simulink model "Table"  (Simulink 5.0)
settings: Solver=FixedStepDiscrete  SolverMode=SingleTasking  StartTime=0.0  StopTime=inf  FixedStep=samplePeriod  RelTol=1e-3  AbsTol=1e-6
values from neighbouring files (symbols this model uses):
  accelCalib = ones(1, size(ra_t, 2)) * 7848.0    [TableInit.m]
  actParamsX = [bulkModulus    * pressCanon,    [TableInit.m]
  actParamsY = [bulkModulus    * pressCanon,    [TableInit.m]
  actParamsZ = [bulkModulus    * pressCanon,    [TableInit.m]
  aHome = zeros(1, nAct)    [TableInit.m]    (also in displA2T.m = positT2A([0, 0, 0, 0, 0, 0], h); displT2A.m = positT2A([0, 0, 0, 0, 0, 0], h))
  bal = [[ 1 -1 -1  1  0  0  0  0]    [TableInit.m]
  displCalib = [300.0 300.0 300.0 300.0 250.0 250.0 250.0 250.0]    [TableInit.m]
  ea_t = zeros(3, nAcc)    [TableInit.m]
  flowCanon = 63090.2    [TableInit.m]    (also in initialize.m)
  forceCalib = [366.5 366.5 366.5 366.5 366.5 366.5 366.5 366.5]    [TableInit.m]
  gasConstant = 1.8    [TableInit.m]    (also in initialize.m)
  gee = 0    [TableInit.m]    (also in initialize.m = geeCanon / linAccelCanon * ~isempty(find(dof==3)))
  inertia = [Ixx 0 0; 0 Iyy 0; 0 0 Izz]    [TableInit.m]    (also in initialize.m = inertia + inertiaP2Q([0 0 0], massA(i), cgA(:,i)-cg,  						)
  inertiaCanon = 0.1130    (= 0.113)    [TableInit.m]    (also in initialize.m = 0.00029264264)
  linAccelCanon = 9.8    [TableInit.m]    (also in accelA2T.m = h(11); accelT2A.m = h(11); Test.m = 9800; initialize.m = 9810)
  linVelocCanon = 10.0    (= 10)    [TableInit.m]    (also in Test.m; initialize.m = 1000)
  mass = 17300    [TableInit.m]    (also in initialize.m = ones(3, 1) * (sum(massA) + massT + massS))
  massCanon = 0.4535924e-06    (= 4.535924e-07)    [TableInit.m]    (also in initialize.m)
  maxDispl = zeros(1, nAct)    [TableInit.m]    (also in initialize.m = max(abs(maxDispl), abs(minDispl)))
  maxOilVolume = volume * (1 - (precharge/supplyPress)^(1/gasConstant))    (= 316.850998915)    [TableInit.m]
  precharge = 1916    [TableInit.m]    (also in initialize.m = 2000)
  pumpFlow = 1.0e10    (= 10000000000)    [TableInit.m]    (also in initialize.m)
  ra_t = [-1600.00   233.10  -233.10  1600.00 -1000.00  1000.00 -1000.00  1000.00        0    [TableInit.m]    (also in accelA2T.m = [  0   0   0 -h7  h7   0 -h7 -h7  h7  h7   0;          -h7  ; accelT2A.m = [  0   0   0 -h7  h7   0 -h7 -h7  h7  h7   0;          -h7  )
  rb_w = [-1525.00  3683.70 -3683.70  1525.00 -1000.00  1000.00 -1000.00  1000.00    [TableInit.m]    (also in positT2A.m = [-h1 -h5  h5  h1 -h1 -h1  h1  h1;           h5 -h1  h1 -h5  ; animation.m = self.R * rb_w)
  returnPress = 50    [TableInit.m]    (also in initialize.m)
  rgt = -rtg    [TableInit.m]
  rotAccelCanon = 1    [TableInit.m]    (also in accelA2T.m = h(14); accelT2A.m = h(14); Test.m; initialize.m = 0.0174532925199)
  rotForceCanon = 1000    [TableInit.m]    (also in forceA2T.m = h(15); Test.m; initialize.m)
  rotVelocCanon = 1    [TableInit.m]    (also in accelA2T.m = h(13); accelT2A.m = h(13); Test.m; initialize.m = 0.0174532925199)
  rt_t = [-1525.00  1214.70 -1214.70  1525.00 -1000.00  1000.00 -1000.00  1000.00    [TableInit.m]    (also in positT2A.m = [-h1    -h4-sh  h4+sh  h1    -h1    -h1     h1     h1;      )
  rtg = [0 0 cg]    [TableInit.m]    (also in initialize.m = cg)
  rtx_t = [rt_t topPlane.topLeft(:)  topPlane.topRight(:)                        topPlane.botRight(:) topPlane.botLeft(:)                         midPlane.topLeft(:)  midPlane.topRight(:)                        midPlane.botRight(:) midPlane.botLeft(:)                         botPlane.topLeft(:)  botPlane.topRight(:)                        botPlane.botRight(:) botPlane.botLeft(:)]    [TableInit.m]
  samplePeriod = 1/1024    (= 0.0009765625)    [TableInit.m]    (also in viewer.m = eval(getHeaderValue(header, 'DELTA_T')); initialize.m = 0.00048828125)
  volume = 1437    [TableInit.m]    (also in quake.m = volume / 231.0; initialize.m = 160)
  volumeCanon = 3785412.0    (= 3785412)    [TableInit.m]    (also in initialize.m)
undefined symbols (not defined in the file or in its folder): magnitude
libraries: aerospace x41, simulink x19, simulink_extras x1

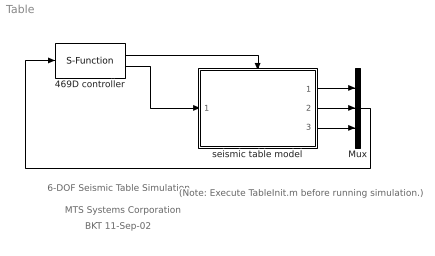
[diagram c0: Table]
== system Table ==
  note: BKT 11-Sep-02
  note: MTS Systems Corporation
  note: 6-DOF Seismic Table Simulation
  note: (Note: Execute TableInit.m before running simulation.)
  469D controller : S-Function  FunctionName=mtsConnect  Parameters='127.0.0.1',5002,nAct+nAct+nAcc,nAct
  Mux : Mux  Inputs=3
  seismic table model : Subsystem  TreatAsAtomicUnit=on
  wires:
  seismic table model/1(displ) -> Mux/1
  seismic table model/2(force) -> Mux/2
  seismic table model/3(accel) -> Mux/3
  Mux/1 -> 469D controller/1
  469D controller/2 -> seismic table model/1(valve cmd)
  469D controller/1 -> seismic table model/Trigger

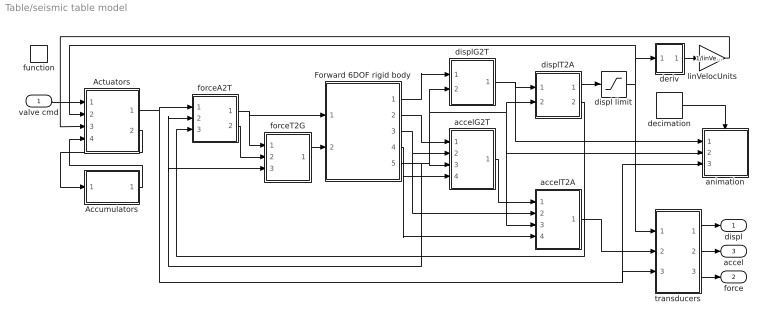
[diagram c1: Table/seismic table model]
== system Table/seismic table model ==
  valve cmd : Inport
  function : TriggerPort  TriggerType=function-call
  Accumulators : Subsystem
  Actuators : Subsystem
  Forward 6DOF rigid body : Subsystem
  accelG2T : Subsystem
  accelT2A : Subsystem
  animation : Subsystem  TreatAsAtomicUnit=on  mask{type=2, azim=-37.5, elev=15}
      mask prompts: type "Drawing type (0: none, 1: wire frame, 2: solid)"; azim "View azimuth (degrees)"; elev "View elevation (degrees)"
  decimation : DiscretePulseGenerator  Period=64  SampleTime=-1
  deriv : Subsystem  mask{T=samplePeriod}
      mask prompts: T "Sample period (sec)"
  displ limit : Saturate  UpperLimit=maxDispl(:)  LowerLimit=-maxDispl(:)
  displG2T : Subsystem
  displT2A : Subsystem
  forceA2T : Subsystem
  forceT2G : Subsystem
  linVelocUnits : Gain  Gain=1/linVelocCanon
  transducers : Subsystem
  displ : Outport
  force : Outport  Port=2
  accel : Outport  Port=3
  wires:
  valve cmd/1 -> Actuators/1(cmds)
  displT2A/1(out) -> displ limit/1
  deriv/1(out) -> linVelocUnits/1
  displT2A/2(dir) -> forceA2T/3(dir)
  Actuators/1(force) -> forceA2T/1(inp), transducers/3(force), animation/3(Fact)
  forceA2T/1(xyz) -> forceT2G/1(xyz), Forward 6DOF rigid body/1(Fxyz)
  displG2T/1(out) -> displT2A/1(xyz), animation/1(xyz)
  Forward 6DOF rigid body/5(DCM) -> displT2A/2(DCM), accelT2A/3(DCM), animation/2(DCM), displG2T/2(DCM), accelG2T/3(DCM), forceA2T/2(DCM), forceT2G/3(DCM)
  accelG2T/1(out) -> accelT2A/1(xyz)
  forceA2T/2(rpw) -> forceT2G/2(rpw)
  forceT2G/1(out) -> Forward 6DOF rigid body/2(Mxyz)
  displ limit/1 -> Actuators/2(displ), deriv/1(inp), transducers/1(displ)
  Forward 6DOF rigid body/1(xyz) -> displG2T/1(xyz)
  Forward 6DOF rigid body/4(rot veloc) -> accelT2A/4(rot veloc), accelG2T/4(rot veloc)
  Forward 6DOF rigid body/3(rot accel) -> accelT2A/2(rpw), accelG2T/2(rpw)
  Forward 6DOF rigid body/2(lin accel) -> accelG2T/1(xyz)
  linVelocUnits/1 -> Actuators/3(veloc)
  Actuators/2(flow) -> Accumulators/1(flow)
  Accumulators/1(press) -> Actuators/4(press)
  accelT2A/1(out) -> transducers/2(accel)
  transducers/1(out1) -> displ/1
  transducers/2(out2) -> accel/1
  transducers/3(out3) -> force/1
  decimation/1 -> animation/Trigger

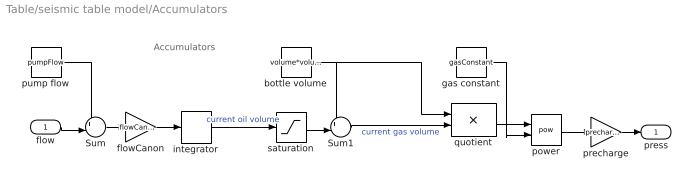
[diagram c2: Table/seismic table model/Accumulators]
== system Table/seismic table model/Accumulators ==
  note: Accumulators
  flow : Inport
  Sum : Sum  Inputs=+-|
  Sum1 : Sum  Inputs=+-|
  bottle volume : Constant  Value=volume*volumeCanon
  flowCanon : Gain  Gain=flowCanon
  gas constant : Constant  Value=gasConstant
  integrator : DiscreteIntegrator  InitialCondition=volume * (1 - (precharge/3000)^(1/gasConstant)) * 231  SampleTime=-1
  power : Math  Operator=pow
  precharge : Gain  Gain=precharge
  pump flow : Constant  Value=pumpFlow
  quotient : Product  Inputs=*/
  saturation : Saturate  UpperLimit=maxOilVolume*volumeCanon  LowerLimit=0
  press : Outport
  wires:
  pump flow/1 -> Sum/1
  Sum/1 -> flowCanon/1
  bottle volume/1 -> Sum1/1, quotient/1
  saturation/1 -> Sum1/2
  gas constant/1 -> power/2
  power/1 -> precharge/1
  precharge/1 -> press/1
  Sum1/1 -> quotient/2  "current gas volume"
  quotient/1 -> power/1
  integrator/1 -> saturation/1  "current oil volume"
  flow/1 -> Sum/2
  flowCanon/1 -> integrator/1

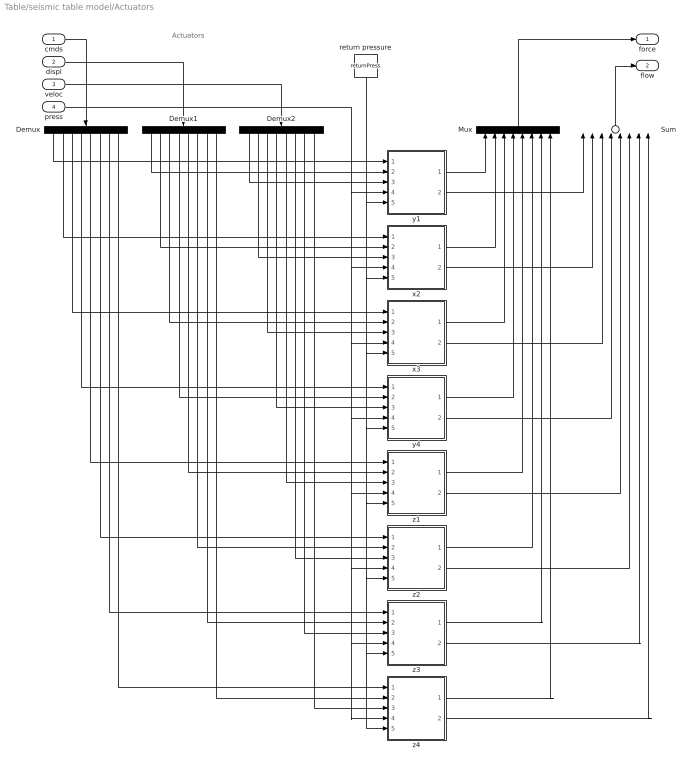
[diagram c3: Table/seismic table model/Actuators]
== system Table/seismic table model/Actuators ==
  note: Actuators
  cmds : Inport
  displ : Inport  Port=2
  veloc : Inport  Port=3
  press : Inport  Port=4
  Demux : Demux  Orientation=down  Outputs=8
  Demux1 : Demux  Orientation=down  Outputs=8
  Demux2 : Demux  Orientation=down  Outputs=8
  Mux : Mux  Orientation=up  Inputs=8
  Sum : Sum  Orientation=up  Inputs=8
  return pressure : Constant  Orientation=down  Value=returnPress
  x2 : Subsystem  mask(Inverse Actuator){params=actParamsX}
      mask prompts: params "Parameter vector"
  x3 : Subsystem  mask(Inverse Actuator){params=actParamsX}
      mask prompts: params "Parameter vector"
  y1 : Subsystem  mask(Inverse Actuator){params=actParamsY}
      mask prompts: params "Parameter vector"
  y4 : Subsystem  mask(Inverse Actuator){params=actParamsY}
      mask prompts: params "Parameter vector"
  z1 : Subsystem  mask(Inverse Actuator){params=actParamsZ}
      mask prompts: params "Parameter vector"
  z2 : Subsystem  mask(Inverse Actuator){params=actParamsZ}
      mask prompts: params "Parameter vector"
  z3 : Subsystem  mask(Inverse Actuator){params=actParamsZ}
      mask prompts: params "Parameter vector"
  z4 : Subsystem  mask(Inverse Actuator){params=actParamsZ}
      mask prompts: params "Parameter vector"
  force : Outport
  flow : Outport  Port=2
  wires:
  cmds/1 -> Demux/1
  displ/1 -> Demux1/1
  Demux/1 -> y1/1(cmd)
  Demux/2 -> x2/1(cmd)
  Demux1/1 -> y1/2(displ)
  Demux2/1 -> y1/3(veloc)
  Demux1/2 -> x2/2(displ)
  Demux2/2 -> x2/3(veloc)
  Demux/3 -> x3/1(cmd)
  Demux1/3 -> x3/2(displ)
  Demux2/3 -> x3/3(veloc)
  Demux/4 -> y4/1(cmd)
  Demux1/4 -> y4/2(displ)
  Demux2/4 -> y4/3(veloc)
  Demux/5 -> z1/1(cmd)
  Demux1/5 -> z1/2(displ)
  Demux2/5 -> z1/3(veloc)
  Demux/6 -> z2/1(cmd)
  Demux1/6 -> z2/2(displ)
  Demux2/6 -> z2/3(veloc)
  Demux/7 -> z3/1(cmd)
  Demux1/7 -> z3/2(displ)
  Demux2/7 -> z3/3(veloc)
  Demux/8 -> z4/1(cmd)
  Demux1/8 -> z4/2(displ)
  Demux2/8 -> z4/3(veloc)
  y1/1(force) -> Mux/1
  x2/1(force) -> Mux/2
  x3/1(force) -> Mux/3
  y4/1(force) -> Mux/4
  Mux/1 -> force/1
  z1/1(force) -> Mux/5
  z2/1(force) -> Mux/6
  z3/1(force) -> Mux/7
  z4/1(force) -> Mux/8
  veloc/1 -> Demux2/1
  press/1 -> z3/4(spl press), z4/4(spl press), z2/4(spl press), z1/4(spl press), y4/4(spl press), x3/4(spl press), x2/4(spl press), y1/4(spl press)
  return pressure/1 -> z3/5(rtn press), z4/5(rtn press), z2/5(rtn press), z1/5(rtn press), y4/5(rtn press), x3/5(rtn press), x2/5(rtn press), y1/5(rtn press)
  Sum/1 -> flow/1
  y1/2(flow) -> Sum/1
  x2/2(flow) -> Sum/2
  x3/2(flow) -> Sum/3
  y4/2(flow) -> Sum/4
  z1/2(flow) -> Sum/5
  z2/2(flow) -> Sum/6
  z3/2(flow) -> Sum/7
  z4/2(flow) -> Sum/8

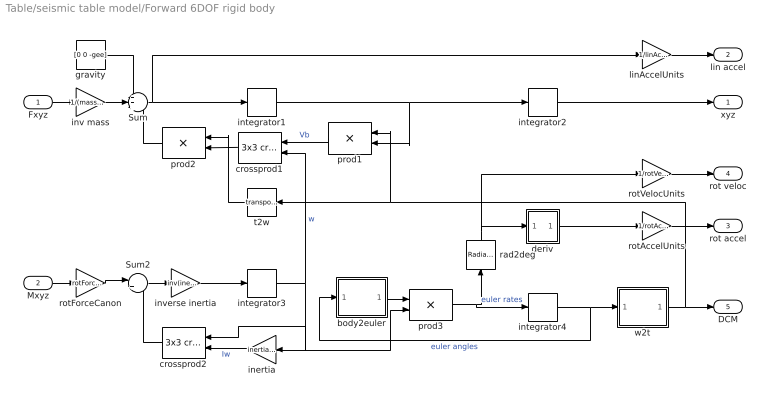
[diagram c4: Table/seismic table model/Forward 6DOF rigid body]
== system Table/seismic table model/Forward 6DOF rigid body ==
  Fxyz : Inport
  Mxyz : Inport  Port=2
  Sum : Sum  Inputs=+++
  Sum2 : Sum  Inputs=|+-
  body2euler : Subsystem
  crossprod1 : aerospace/Axes Transformations/3x3 cross product  Orientation=left
  crossprod2 : aerospace/Axes Transformations/3x3 cross product  Orientation=left
  deriv : Subsystem  mask{T=samplePeriod}
      mask prompts: T "Sample period (sec)"
  gravity : Constant  Value=[0 0 -gee]
  inertia : Gain  Orientation=left  Gain=inertia*inertiaCanon  Multiplication=Matrix(K*u)
  integrator{1..4} (4 alike) : DiscreteIntegrator  SampleTime=-1
  inv mass : Gain  Gain=1/(mass*massCanon)
  inverse inertia : Gain  Gain=inv(inertia*inertiaCanon)  Multiplication=Matrix(K*u)
  linAccelUnits : Gain  Gain=1/linAccelCanon
  prod1 : Product  Orientation=left  Multiplication=Matrix(*)
  prod2 : Product  Orientation=left  Multiplication=Matrix(*)
  prod3 : Product  Multiplication=Matrix(*)
  rad2deg : simulink_extras/Transformations/Radians to Degrees  Orientation=up
  rotAccelUnits : Gain  Gain=1/rotAccelCanon
  rotForceCanon : Gain  Gain=rotForceCanon
  rotVelocUnits : Gain  Gain=1/rotVelocCanon
  t2w : Math  Orientation=left  Operator=transpose
  w2t : Subsystem
  xyz : Outport
  lin accel : Outport  Port=2
  rot accel : Outport  Port=3
  rot veloc : Outport  Port=4
  DCM : Outport  Port=5
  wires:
  inertia/1 -> crossprod2/2  "Iw"
  Sum2/1 -> inverse inertia/1
  integrator3/1 -> inertia/1, crossprod2/1, prod3/2, crossprod1/2  "w"
  integrator1/1 -> prod1/2, integrator2/1
  Mxyz/1 -> rotForceCanon/1
  inverse inertia/1 -> integrator3/1
  body2euler/1(out) -> prod3/1
  prod3/1 -> integrator4/1, rad2deg/1  "euler rates"
  w2t/1(DCM) -> t2w/1, prod1/1, DCM/1
  rotVelocUnits/1 -> rot veloc/1
  rotForceCanon/1 -> Sum2/1
  linAccelUnits/1 -> lin accel/1
  integrator2/1 -> xyz/1
  gravity/1 -> Sum/1
  Fxyz/1 -> inv mass/1
  inv mass/1 -> Sum/2
  Sum/1 -> linAccelUnits/1, integrator1/1
  crossprod1/1 -> prod2/2
  prod2/1 -> Sum/3
  t2w/1 -> prod2/1
  prod1/1 -> crossprod1/1  "Vb"
  rotAccelUnits/1 -> rot accel/1
  integrator4/1 -> w2t/1(rpw), body2euler/1(rpw)  "euler angles"
  deriv/1(out) -> rotAccelUnits/1
  crossprod2/1 -> Sum2/2
  rad2deg/1 -> deriv/1(inp), rotVelocUnits/1

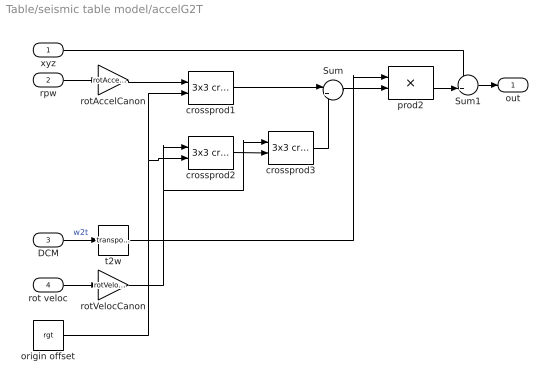
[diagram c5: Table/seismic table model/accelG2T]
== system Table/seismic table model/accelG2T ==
  xyz : Inport
  rpw : Inport  Port=2
  DCM : Inport  Port=3
  rot veloc : Inport  Port=4
  Sum : Sum  Inputs=|++
  Sum1 : Sum  Inputs=++|
  crossprod1 : aerospace/Axes Transformations/3x3 cross product
  crossprod2 : aerospace/Axes Transformations/3x3 cross product
  crossprod3 : aerospace/Axes Transformations/3x3 cross product
  origin offset : Constant  Value=rgt
  prod2 : Product  Multiplication=Matrix(*)
  rotAccelCanon : Gain  Gain=rotAccelCanon*(pi/180)/linAccelCanon
  rotVelocCanon : Gain  Gain=rotVelocCanon*(pi/180)/sqrt(linAccelCanon)
  t2w : Math  Operator=transpose
  out : Outport
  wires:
  rotVelocCanon/1 -> crossprod2/1, crossprod3/1
  DCM/1 -> t2w/1  "w2t"
  rot veloc/1 -> rotVelocCanon/1
  xyz/1 -> Sum1/1
  t2w/1 -> prod2/1
  rpw/1 -> rotAccelCanon/1
  rotAccelCanon/1 -> crossprod1/1
  origin offset/1 -> crossprod2/2, crossprod1/2
  Sum/1 -> prod2/2
  crossprod2/1 -> crossprod3/2
  prod2/1 -> Sum1/2
  Sum1/1 -> out/1
  crossprod3/1 -> Sum/2
  crossprod1/1 -> Sum/1

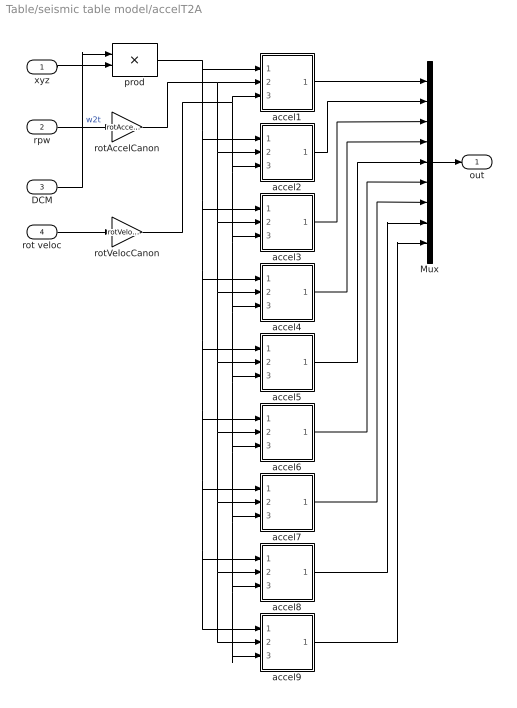
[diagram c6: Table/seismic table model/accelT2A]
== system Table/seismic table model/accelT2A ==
  xyz : Inport
  rpw : Inport  Port=2
  DCM : Inport  Port=3
  rot veloc : Inport  Port=4
  Mux : Mux  Inputs=9
  accel1 : Subsystem  mask{id=1}
      mask prompts: id "Accelerometer number"
  accel2 : Subsystem  mask{id=2}
      mask prompts: id "Accelerometer number"
  accel3 : Subsystem  mask{id=3}
      mask prompts: id "Accelerometer number"
  accel4 : Subsystem  mask{id=4}
      mask prompts: id "Accelerometer number"
  accel5 : Subsystem  mask{id=5}
      mask prompts: id "Accelerometer number"
  accel6 : Subsystem  mask{id=6}
      mask prompts: id "Accelerometer number"
  accel7 : Subsystem  mask{id=7}
      mask prompts: id "Accelerometer number"
  accel8 : Subsystem  mask{id=8}
      mask prompts: id "Accelerometer number"
  accel9 : Subsystem  mask{id=9}
      mask prompts: id "Accelerometer number"
  prod : Product  Multiplication=Matrix(*)
  rotAccelCanon : Gain  Gain=rotAccelCanon*(pi/180)/linAccelCanon
  rotVelocCanon : Gain  Gain=rotVelocCanon*(pi/180)/sqrt(linAccelCanon)
  out : Outport
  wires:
  xyz/1 -> prod/2
  prod/1 -> accel1/1(linacc), accel8/1(linacc), accel9/1(linacc), accel7/1(linacc), accel6/1(linacc), accel5/1(linacc), accel4/1(linacc), accel3/1(linacc), accel2/1(linacc)
  rpw/1 -> rotAccelCanon/1
  rot veloc/1 -> rotVelocCanon/1
  DCM/1 -> prod/1  "w2t"
  rotVelocCanon/1 -> accel1/3(rotvel), accel8/3(rotvel), accel9/3(rotvel), accel7/3(rotvel), accel6/3(rotvel), accel5/3(rotvel), accel4/3(rotvel), accel3/3(rotvel), accel2/3(rotvel)
  rotAccelCanon/1 -> accel1/2(rotacc), accel8/2(rotacc), accel9/2(rotacc), accel7/2(rotacc), accel6/2(rotacc), accel5/2(rotacc), accel4/2(rotacc), accel3/2(rotacc), accel2/2(rotacc)
  accel1/1(out) -> Mux/1
  accel2/1(out) -> Mux/2
  Mux/1 -> out/1
  accel9/1(out) -> Mux/9
  accel8/1(out) -> Mux/8
  accel7/1(out) -> Mux/7
  accel6/1(out) -> Mux/6
  accel5/1(out) -> Mux/5
  accel4/1(out) -> Mux/4
  accel3/1(out) -> Mux/3

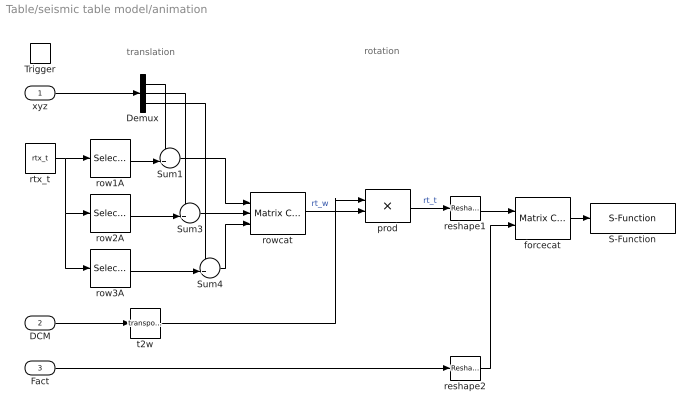
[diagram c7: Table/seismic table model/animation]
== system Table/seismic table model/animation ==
  note: translation
  note: rotation
  xyz : Inport
  DCM : Inport  Port=2
  Fact : Inport  Port=3
  Trigger : TriggerPort
  Demux : Demux  Outputs=3
  S-Function : S-Function  FunctionName=tableAnimation  Parameters=type, rb_w,zmax,fmax,lines,faces,cmap,azim,elev
  Sum1 : Sum  Inputs=-+|
  Sum3 : Sum  Inputs=-+|
  Sum4 : Sum  Inputs=-+|
  forcecat : simulink/Math Operations/Matrix Concatenation  numInports=2  catMethod=Vertical
  prod : Product  Multiplication=Matrix(*)
  reshape1 : simulink/Math Operations/Reshape  OutputDimensionality=1-D array  OutputDimensions=[1,1]
  reshape2 : simulink/Math Operations/Reshape  OutputDimensionality=1-D array  OutputDimensions=[1,1]
  row1A : Selector  InputType=Matrix  Elements=[1 3]  Columns=-1  InputPortWidth=3
  row2A : Selector  InputType=Matrix  Elements=[1 3]  Rows=2  Columns=-1  InputPortWidth=3
  row3A : Selector  InputType=Matrix  Elements=[1 3]  Rows=3  Columns=-1  InputPortWidth=3
  rowcat : simulink/Math Operations/Matrix Concatenation  numInports=3  catMethod=Vertical
  rtx_t : Constant  Value=rtx_t
  t2w : Math  Operator=transpose
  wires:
  DCM/1 -> t2w/1
  xyz/1 -> Demux/1
  row1A/1 -> Sum1/2
  Demux/1 -> Sum1/1
  row2A/1 -> Sum3/2
  row3A/1 -> Sum4/2
  Demux/2 -> Sum3/1
  Demux/3 -> Sum4/1
  Sum3/1 -> rowcat/2
  Sum1/1 -> rowcat/1
  Sum4/1 -> rowcat/3
  t2w/1 -> prod/1
  rtx_t/1 -> row1A/1, row2A/1, row3A/1
  rowcat/1 -> prod/2  "rt_w"
  prod/1 -> reshape1/1  "rt_t"
  Fact/1 -> reshape2/1
  reshape1/1 -> forcecat/1
  forcecat/1 -> S-Function/1
  reshape2/1 -> forcecat/2

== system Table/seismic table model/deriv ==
  inp : Inport
  1/T : Gain  Gain=1/T
  Sum : Sum  Inputs=|+-
  Unit Delay : UnitDelay  SampleTime=-1
  out : Outport
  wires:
  1/T/1 -> out/1
  Sum/1 -> 1/T/1
  Unit Delay/1 -> Sum/2
  inp/1 -> Unit Delay/1, Sum/1

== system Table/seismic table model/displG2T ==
  xyz : Inport
  DCM : Inport  Port=2
  Sum1 : Sum  Inputs=+-+
  origin offset : Constant  Value=rgt
  prod : Product  Multiplication=Matrix(*)
  out : Outport
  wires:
  DCM/1 -> prod/1
  origin offset/1 -> prod/2, Sum1/3
  xyz/1 -> Sum1/1
  prod/1 -> Sum1/2
  Sum1/1 -> out/1

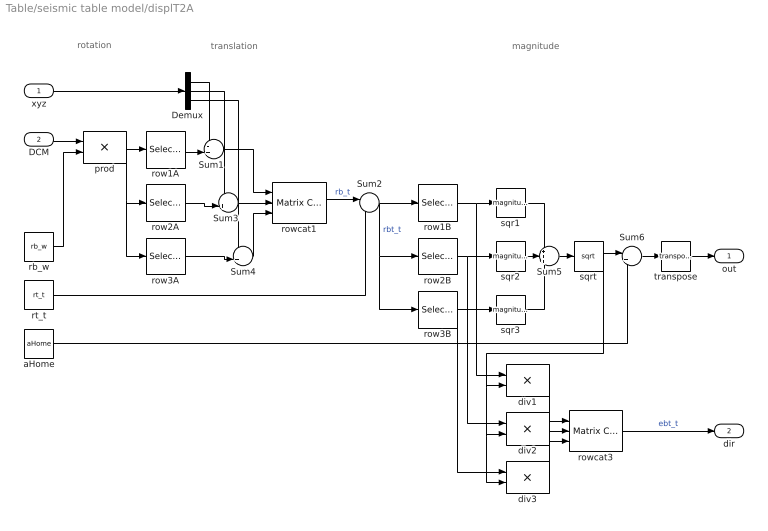
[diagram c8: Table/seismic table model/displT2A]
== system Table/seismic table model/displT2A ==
  note: rotation
  note: magnitude
  note: translation
  xyz : Inport
  DCM : Inport  Port=2
  Demux : Demux  Outputs=3
  Sum1 : Sum  Inputs=-+|
  Sum2 : Sum  Inputs=|-+
  Sum3 : Sum  Inputs=-+|
  Sum4 : Sum  Inputs=-+|
  Sum5 : Sum  Inputs=+++
  Sum6 : Sum  Inputs=|+-
  aHome : Constant  Value=aHome
  div1 : Product  Inputs=*/
  div2 : Product  Inputs=*/
  div3 : Product  Inputs=*/
  prod : Product  Multiplication=Matrix(*)
  rb_w : Constant  Value=rb_w
  row1A : Selector  InputType=Matrix  Elements=[1 3]  Columns=-1  InputPortWidth=3
  row1B : Selector  InputType=Matrix  Elements=[1 3]  Columns=-1  InputPortWidth=3
  row2A : Selector  InputType=Matrix  Elements=[1 3]  Rows=2  Columns=-1  InputPortWidth=3
  row2B : Selector  InputType=Matrix  Elements=[1 3]  Rows=2  Columns=-1  InputPortWidth=3
  row3A : Selector  InputType=Matrix  Elements=[1 3]  Rows=3  Columns=-1  InputPortWidth=3
  row3B : Selector  InputType=Matrix  Elements=[1 3]  Rows=3  Columns=-1  InputPortWidth=3
  rowcat1 : simulink/Math Operations/Matrix Concatenation  numInports=3  catMethod=Vertical
  rowcat3 : simulink/Math Operations/Matrix Concatenation  numInports=3  catMethod=Vertical
  rt_t : Constant  Value=rt_t
  sqr1 : Math  Operator=magnitude^2
  sqr2 : Math  Operator=magnitude^2
  sqr3 : Math  Operator=magnitude^2
  sqrt : Math  Operator=sqrt
  transpose : Math  Operator=transpose
  out : Outport
  dir : Outport  Port=2
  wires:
  rb_w/1 -> prod/2
  prod/1 -> row1A/1, row3A/1, row2A/1
  xyz/1 -> Demux/1
  row1A/1 -> Sum1/2
  Demux/1 -> Sum1/1
  row2A/1 -> Sum3/2
  row3A/1 -> Sum4/2
  Demux/2 -> Sum3/1
  Demux/3 -> Sum4/1
  Sum3/1 -> rowcat1/2
  Sum1/1 -> rowcat1/1
  Sum4/1 -> rowcat1/3
  rt_t/1 -> Sum2/2
  row2B/1 -> sqr2/1, div2/1
  row1B/1 -> sqr1/1, div1/1
  row3B/1 -> sqr3/1, div3/1
  Sum5/1 -> sqrt/1
  aHome/1 -> Sum6/2
  sqrt/1 -> Sum6/1, div1/2, div2/2, div3/2
  rowcat1/1 -> Sum2/1  "rb_t"
  Sum2/1 -> row3B/1, row2B/1, row1B/1  "rbt_t"
  sqr1/1 -> Sum5/1
  sqr2/1 -> Sum5/2
  sqr3/1 -> Sum5/3
  rowcat3/1 -> dir/1  "ebt_t"
  div1/1 -> rowcat3/1
  div2/1 -> rowcat3/2
  div3/1 -> rowcat3/3
  DCM/1 -> prod/1
  Sum6/1 -> transpose/1
  transpose/1 -> out/1

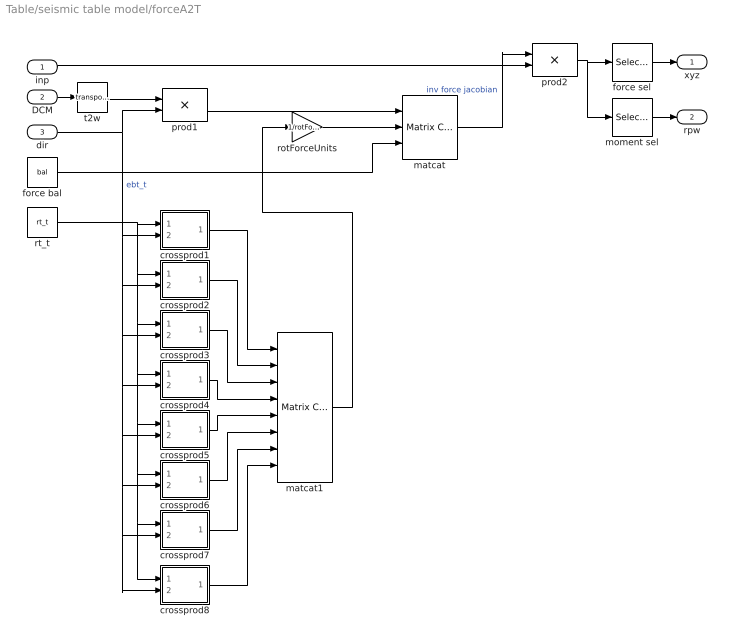
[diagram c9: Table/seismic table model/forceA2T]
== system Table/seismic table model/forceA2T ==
  inp : Inport
  DCM : Inport  Port=2
  dir : Inport  Port=3
  crossprod1 : Subsystem  mask{id=1}
      mask prompts: id "Actuator number"
  crossprod2 : Subsystem  mask{id=2}
      mask prompts: id "Actuator number"
  crossprod3 : Subsystem  mask{id=3}
      mask prompts: id "Actuator number"
  crossprod4 : Subsystem  mask{id=4}
      mask prompts: id "Actuator number"
  crossprod5 : Subsystem  mask{id=5}
      mask prompts: id "Actuator number"
  crossprod6 : Subsystem  mask{id=6}
      mask prompts: id "Actuator number"
  crossprod7 : Subsystem  mask{id=7}
      mask prompts: id "Actuator number"
  crossprod8 : Subsystem  mask{id=8}
      mask prompts: id "Actuator number"
  force bal : Constant  Value=bal
  force sel : Selector  Elements=[1 2 3]
  matcat : simulink/Math Operations/Matrix Concatenation  numInports=3  catMethod=Vertical
  matcat1 : simulink/Math Operations/Matrix Concatenation  numInports=8  catMethod=Horizontal
  moment sel : Selector  Elements=[4 5 6]
  prod1 : Product  Multiplication=Matrix(*)
  prod2 : Product  Multiplication=Matrix(*)
  rotForceUnits : Gain  Gain=1/rotForceCanon
  rt_t : Constant  Value=rt_t
  t2w : Math  Operator=transpose
  xyz : Outport
  rpw : Outport  Port=2
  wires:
  rotForceUnits/1 -> matcat/2
  matcat/1 -> prod2/1  "inv force jacobian"
  force sel/1 -> xyz/1
  moment sel/1 -> rpw/1
  DCM/1 -> t2w/1
  dir/1 -> prod1/2, crossprod1/2(B), crossprod7/2(B), crossprod8/2(B), crossprod6/2(B), crossprod5/2(B), crossprod4/2(B), crossprod3/2(B), crossprod2/2(B)  "ebt_t"
  prod1/1 -> matcat/1
  rt_t/1 -> crossprod1/1(A), crossprod7/1(A), crossprod8/1(A), crossprod6/1(A), crossprod5/1(A), crossprod4/1(A), crossprod3/1(A), crossprod2/1(A)
  matcat1/1 -> rotForceUnits/1
  crossprod1/1(AxB) -> matcat1/1
  crossprod2/1(AxB) -> matcat1/2
  crossprod3/1(AxB) -> matcat1/3
  crossprod4/1(AxB) -> matcat1/4
  crossprod5/1(AxB) -> matcat1/5
  crossprod6/1(AxB) -> matcat1/6
  crossprod7/1(AxB) -> matcat1/7
  crossprod8/1(AxB) -> matcat1/8
  inp/1 -> prod2/2
  t2w/1 -> prod1/1
  prod2/1 -> force sel/1, moment sel/1
  force bal/1 -> matcat/3

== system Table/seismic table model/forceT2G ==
  xyz : Inport
  rpw : Inport  Port=2
  DCM : Inport  Port=3
  Sum : Sum  Inputs=++|
  crossprod : aerospace/Axes Transformations/3x3 cross product
  origin offset : Constant  Value=rtg
  prod : Product  Multiplication=Matrix(*)
  rotForceUnits : Gain  Gain=1/rotForceCanon
  out : Outport
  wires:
  rpw/1 -> Sum/2
  Sum/1 -> out/1
  crossprod/1 -> rotForceUnits/1
  rotForceUnits/1 -> Sum/1
  xyz/1 -> prod/2
  DCM/1 -> prod/1
  prod/1 -> crossprod/1
  origin offset/1 -> crossprod/2

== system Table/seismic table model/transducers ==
  displ : Inport
  accel : Inport  Port=2
  force : Inport  Port=3
  accel egu to volts : Constant  Value=10./accelCalib
  displ egu to volts : Constant  Value=10./displCalib
  force egu to volts : Constant  Value=10./forceCalib
  prod1 : Product
  prod2 : Product
  prod3 : Product
  out1 : Outport
  out2 : Outport  Port=2
  out3 : Outport  Port=3
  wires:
  displ/1 -> prod1/1
  force/1 -> prod3/1
  accel/1 -> prod2/1
  prod1/1 -> out1/1
  prod2/1 -> out2/1
  prod3/1 -> out3/1
  displ egu to volts/1 -> prod1/2
  accel egu to volts/1 -> prod2/2
  force egu to volts/1 -> prod3/2

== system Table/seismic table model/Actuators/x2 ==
  note: Auxiliary diagnostic output vector: 1: valve opening 2: C1 pressure 3: C2 pressure 4: delta pressure 5: force 6: velocity 7: C1 flow 8: C2 flow 9: total flow 10: kinematic flow 11: compressibility flow 12: leakage flow
  note: Parameter vector: 1: oil bulk modulus (force/displ^2) 2: servovalve natural frequency (Hz) 3: servovalve damping ratio 4: servovalve overlap 5: rated pressure (force/displ^2) 6: flow at rated pressure (displ^3/sec) 7: actuator piston area 1 (displ^2) 8: actuator piston area 2 (displ^2) 9: actuator usable length (displ) 10: actuator endcap length (displ) 11: actuator parasitic damping factor 12: cross-chamber leakage factor (flow/press) 13: sample period (sec) Conversion factors used for converting signals from external (user) to internal (canonical) units: 14: displacement 15: velocity 16: force 17: pressure 18: flow
  cmd : Inport
  displ : Inport  Port=2
  veloc : Inport  Port=3
  spl press : Inport  Port=4
  rtn press : Inport  Port=5
  abs : Abs
  actuator : S-Function  FunctionName=actuator  Parameters=params
  total flow sel : Selector  Elements=9  InputPortWidth=12
  force : Outport
  flow : Outport  Port=2
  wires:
  abs/1 -> flow/1
  total flow sel/1 -> abs/1
  actuator/2 -> total flow sel/1
  veloc/1 -> actuator/3
  displ/1 -> actuator/2
  actuator/1 -> force/1
  cmd/1 -> actuator/1
  rtn press/1 -> actuator/5
  spl press/1 -> actuator/4

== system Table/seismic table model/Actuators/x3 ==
  note: Parameter vector: 1: oil bulk modulus (force/displ^2) 2: servovalve natural frequency (Hz) 3: servovalve damping ratio 4: servovalve overlap 5: rated pressure (force/displ^2) 6: flow at rated pressure (displ^3/sec) 7: actuator piston area 1 (displ^2) 8: actuator piston area 2 (displ^2) 9: actuator usable length (displ) 10: actuator endcap length (displ) 11: actuator parasitic damping factor 12: cross-chamber leakage factor (flow/press) 13: sample period (sec) Conversion factors used for converting signals from external (user) to internal (canonical) units: 14: displacement 15: velocity 16: force 17: pressure 18: flow
  note: Auxiliary diagnostic output vector: 1: valve opening 2: C1 pressure 3: C2 pressure 4: delta pressure 5: force 6: velocity 7: C1 flow 8: C2 flow 9: total flow 10: kinematic flow 11: compressibility flow 12: leakage flow
  cmd : Inport
  displ : Inport  Port=2
  veloc : Inport  Port=3
  spl press : Inport  Port=4
  rtn press : Inport  Port=5
  abs : Abs
  actuator : S-Function  FunctionName=actuator  Parameters=params
  total flow sel : Selector  Elements=9  InputPortWidth=12
  force : Outport
  flow : Outport  Port=2
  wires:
  spl press/1 -> actuator/4
  rtn press/1 -> actuator/5
  cmd/1 -> actuator/1
  actuator/1 -> force/1
  displ/1 -> actuator/2
  veloc/1 -> actuator/3
  actuator/2 -> total flow sel/1
  total flow sel/1 -> abs/1
  abs/1 -> flow/1

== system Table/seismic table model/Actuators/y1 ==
  note: Parameter vector: 1: oil bulk modulus (force/displ^2) 2: servovalve natural frequency (Hz) 3: servovalve damping ratio 4: servovalve overlap 5: rated pressure (force/displ^2) 6: flow at rated pressure (displ^3/sec) 7: actuator piston area 1 (displ^2) 8: actuator piston area 2 (displ^2) 9: actuator usable length (displ) 10: actuator endcap length (displ) 11: actuator parasitic damping factor 12: cross-chamber leakage factor (flow/press) 13: sample period (sec) Conversion factors used for converting signals from external (user) to internal (canonical) units: 14: displacement 15: velocity 16: force 17: pressure 18: flow
  note: Auxiliary diagnostic output vector: 1: valve opening 2: C1 pressure 3: C2 pressure 4: delta pressure 5: force 6: velocity 7: C1 flow 8: C2 flow 9: total flow 10: kinematic flow 11: compressibility flow 12: leakage flow
  cmd : Inport
  displ : Inport  Port=2
  veloc : Inport  Port=3
  spl press : Inport  Port=4
  rtn press : Inport  Port=5
  abs : Abs
  actuator : S-Function  FunctionName=actuator  Parameters=params
  total flow sel : Selector  Elements=9  InputPortWidth=12
  force : Outport
  flow : Outport  Port=2
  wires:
  spl press/1 -> actuator/4
  rtn press/1 -> actuator/5
  cmd/1 -> actuator/1
  actuator/1 -> force/1
  displ/1 -> actuator/2
  veloc/1 -> actuator/3
  actuator/2 -> total flow sel/1
  total flow sel/1 -> abs/1
  abs/1 -> flow/1

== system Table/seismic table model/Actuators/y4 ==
  note: Auxiliary diagnostic output vector: 1: valve opening 2: C1 pressure 3: C2 pressure 4: delta pressure 5: force 6: velocity 7: C1 flow 8: C2 flow 9: total flow 10: kinematic flow 11: compressibility flow 12: leakage flow
  note: Parameter vector: 1: oil bulk modulus (force/displ^2) 2: servovalve natural frequency (Hz) 3: servovalve damping ratio 4: servovalve overlap 5: rated pressure (force/displ^2) 6: flow at rated pressure (displ^3/sec) 7: actuator piston area 1 (displ^2) 8: actuator piston area 2 (displ^2) 9: actuator usable length (displ) 10: actuator endcap length (displ) 11: actuator parasitic damping factor 12: cross-chamber leakage factor (flow/press) 13: sample period (sec) Conversion factors used for converting signals from external (user) to internal (canonical) units: 14: displacement 15: velocity 16: force 17: pressure 18: flow
  cmd : Inport
  displ : Inport  Port=2
  veloc : Inport  Port=3
  spl press : Inport  Port=4
  rtn press : Inport  Port=5
  abs : Abs
  actuator : S-Function  FunctionName=actuator  Parameters=params
  total flow sel : Selector  Elements=9  InputPortWidth=12
  force : Outport
  flow : Outport  Port=2
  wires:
  abs/1 -> flow/1
  total flow sel/1 -> abs/1
  actuator/2 -> total flow sel/1
  veloc/1 -> actuator/3
  displ/1 -> actuator/2
  actuator/1 -> force/1
  cmd/1 -> actuator/1
  rtn press/1 -> actuator/5
  spl press/1 -> actuator/4

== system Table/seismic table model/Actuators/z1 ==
  note: Parameter vector: 1: oil bulk modulus (force/displ^2) 2: servovalve natural frequency (Hz) 3: servovalve damping ratio 4: servovalve overlap 5: rated pressure (force/displ^2) 6: flow at rated pressure (displ^3/sec) 7: actuator piston area 1 (displ^2) 8: actuator piston area 2 (displ^2) 9: actuator usable length (displ) 10: actuator endcap length (displ) 11: actuator parasitic damping factor 12: cross-chamber leakage factor (flow/press) 13: sample period (sec) Conversion factors used for converting signals from external (user) to internal (canonical) units: 14: displacement 15: velocity 16: force 17: pressure 18: flow
  note: Auxiliary diagnostic output vector: 1: valve opening 2: C1 pressure 3: C2 pressure 4: delta pressure 5: force 6: velocity 7: C1 flow 8: C2 flow 9: total flow 10: kinematic flow 11: compressibility flow 12: leakage flow
  cmd : Inport
  displ : Inport  Port=2
  veloc : Inport  Port=3
  spl press : Inport  Port=4
  rtn press : Inport  Port=5
  abs : Abs
  actuator : S-Function  FunctionName=actuator  Parameters=params
  total flow sel : Selector  Elements=9  InputPortWidth=12
  force : Outport
  flow : Outport  Port=2
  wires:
  spl press/1 -> actuator/4
  rtn press/1 -> actuator/5
  cmd/1 -> actuator/1
  actuator/1 -> force/1
  displ/1 -> actuator/2
  veloc/1 -> actuator/3
  actuator/2 -> total flow sel/1
  total flow sel/1 -> abs/1
  abs/1 -> flow/1

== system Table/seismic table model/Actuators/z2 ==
  note: Auxiliary diagnostic output vector: 1: valve opening 2: C1 pressure 3: C2 pressure 4: delta pressure 5: force 6: velocity 7: C1 flow 8: C2 flow 9: total flow 10: kinematic flow 11: compressibility flow 12: leakage flow
  note: Parameter vector: 1: oil bulk modulus (force/displ^2) 2: servovalve natural frequency (Hz) 3: servovalve damping ratio 4: servovalve overlap 5: rated pressure (force/displ^2) 6: flow at rated pressure (displ^3/sec) 7: actuator piston area 1 (displ^2) 8: actuator piston area 2 (displ^2) 9: actuator usable length (displ) 10: actuator endcap length (displ) 11: actuator parasitic damping factor 12: cross-chamber leakage factor (flow/press) 13: sample period (sec) Conversion factors used for converting signals from external (user) to internal (canonical) units: 14: displacement 15: velocity 16: force 17: pressure 18: flow
  cmd : Inport
  displ : Inport  Port=2
  veloc : Inport  Port=3
  spl press : Inport  Port=4
  rtn press : Inport  Port=5
  abs : Abs
  actuator : S-Function  FunctionName=actuator  Parameters=params
  total flow sel : Selector  Elements=9  InputPortWidth=12
  force : Outport
  flow : Outport  Port=2
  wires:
  abs/1 -> flow/1
  total flow sel/1 -> abs/1
  actuator/2 -> total flow sel/1
  veloc/1 -> actuator/3
  displ/1 -> actuator/2
  actuator/1 -> force/1
  cmd/1 -> actuator/1
  rtn press/1 -> actuator/5
  spl press/1 -> actuator/4

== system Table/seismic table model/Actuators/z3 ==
  note: Parameter vector: 1: oil bulk modulus (force/displ^2) 2: servovalve natural frequency (Hz) 3: servovalve damping ratio 4: servovalve overlap 5: rated pressure (force/displ^2) 6: flow at rated pressure (displ^3/sec) 7: actuator piston area 1 (displ^2) 8: actuator piston area 2 (displ^2) 9: actuator usable length (displ) 10: actuator endcap length (displ) 11: actuator parasitic damping factor 12: cross-chamber leakage factor (flow/press) 13: sample period (sec) Conversion factors used for converting signals from external (user) to internal (canonical) units: 14: displacement 15: velocity 16: force 17: pressure 18: flow
  note: Auxiliary diagnostic output vector: 1: valve opening 2: C1 pressure 3: C2 pressure 4: delta pressure 5: force 6: velocity 7: C1 flow 8: C2 flow 9: total flow 10: kinematic flow 11: compressibility flow 12: leakage flow
  cmd : Inport
  displ : Inport  Port=2
  veloc : Inport  Port=3
  spl press : Inport  Port=4
  rtn press : Inport  Port=5
  abs : Abs
  actuator : S-Function  FunctionName=actuator  Parameters=params
  total flow sel : Selector  Elements=9  InputPortWidth=12
  force : Outport
  flow : Outport  Port=2
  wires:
  spl press/1 -> actuator/4
  rtn press/1 -> actuator/5
  cmd/1 -> actuator/1
  actuator/1 -> force/1
  displ/1 -> actuator/2
  veloc/1 -> actuator/3
  actuator/2 -> total flow sel/1
  total flow sel/1 -> abs/1
  abs/1 -> flow/1

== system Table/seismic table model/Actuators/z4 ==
  note: Auxiliary diagnostic output vector: 1: valve opening 2: C1 pressure 3: C2 pressure 4: delta pressure 5: force 6: velocity 7: C1 flow 8: C2 flow 9: total flow 10: kinematic flow 11: compressibility flow 12: leakage flow
  note: Parameter vector: 1: oil bulk modulus (force/displ^2) 2: servovalve natural frequency (Hz) 3: servovalve damping ratio 4: servovalve overlap 5: rated pressure (force/displ^2) 6: flow at rated pressure (displ^3/sec) 7: actuator piston area 1 (displ^2) 8: actuator piston area 2 (displ^2) 9: actuator usable length (displ) 10: actuator endcap length (displ) 11: actuator parasitic damping factor 12: cross-chamber leakage factor (flow/press) 13: sample period (sec) Conversion factors used for converting signals from external (user) to internal (canonical) units: 14: displacement 15: velocity 16: force 17: pressure 18: flow
  cmd : Inport
  displ : Inport  Port=2
  veloc : Inport  Port=3
  spl press : Inport  Port=4
  rtn press : Inport  Port=5
  abs : Abs
  actuator : S-Function  FunctionName=actuator  Parameters=params
  total flow sel : Selector  Elements=9  InputPortWidth=12
  force : Outport
  flow : Outport  Port=2
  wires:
  abs/1 -> flow/1
  total flow sel/1 -> abs/1
  actuator/2 -> total flow sel/1
  veloc/1 -> actuator/3
  displ/1 -> actuator/2
  actuator/1 -> force/1
  cmd/1 -> actuator/1
  rtn press/1 -> actuator/5
  spl press/1 -> actuator/4

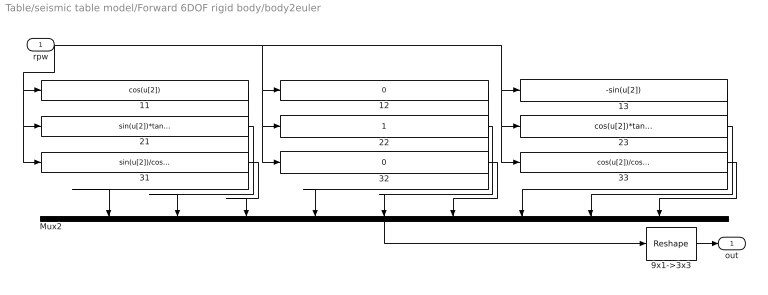
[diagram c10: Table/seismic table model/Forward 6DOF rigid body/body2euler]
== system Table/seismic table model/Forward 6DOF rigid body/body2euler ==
  rpw : Inport
  11 : Fcn  Expr=cos(u[2])
  12 : Fcn  Expr=0
  13 : Fcn  Expr=-sin(u[2])
  21 : Fcn  Expr=sin(u[2])*tan(u[1])
  22 : Fcn  Expr=1
  23 : Fcn  Expr=cos(u[2])*tan(u[1])
  31 : Fcn  Expr=sin(u[2])/cos(u[1])
  32 : Fcn  Expr=0
  33 : Fcn  Expr=cos(u[2])/cos(u[1])
  9x1->3x3 : simulink/Math Operations/Reshape  OutputDimensionality=Customize  OutputDimensions=[3,3]
  Mux2 : Mux  Orientation=down  Inputs=9
  out : Outport
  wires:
  9x1->3x3/1 -> out/1
  11/1 -> Mux2/1
  21/1 -> Mux2/2
  31/1 -> Mux2/3
  rpw/1 -> 31/1, 21/1, 11/1, 32/1, 22/1, 12/1, 33/1, 23/1, 13/1
  12/1 -> Mux2/4
  22/1 -> Mux2/5
  32/1 -> Mux2/6
  Mux2/1 -> 9x1->3x3/1
  13/1 -> Mux2/7
  23/1 -> Mux2/8
  33/1 -> Mux2/9

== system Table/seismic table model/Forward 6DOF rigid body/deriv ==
  inp : Inport
  1/T : Gain  Gain=1/T
  Sum : Sum  Inputs=|+-
  Unit Delay : UnitDelay  SampleTime=-1
  out : Outport
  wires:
  inp/1 -> Sum/1, Unit Delay/1
  Unit Delay/1 -> Sum/2
  Sum/1 -> 1/T/1
  1/T/1 -> out/1

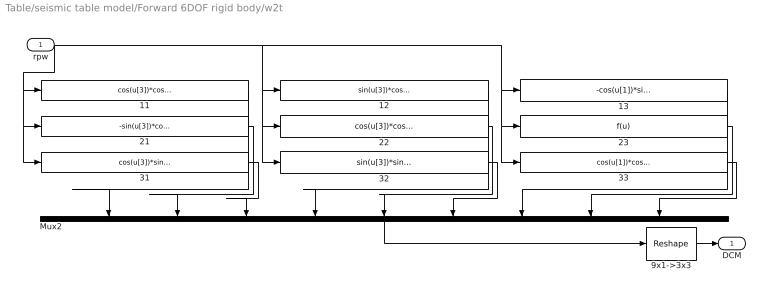
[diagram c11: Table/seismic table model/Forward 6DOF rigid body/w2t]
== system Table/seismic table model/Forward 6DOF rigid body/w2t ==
  rpw : Inport
  11 : Fcn  Expr=cos(u[3])*cos(u[2])-sin(u[3])*sin(u[1])*sin(u[2])
  12 : Fcn  Expr=sin(u[3])*cos(u[2])+cos(u[3])*sin(u[1])*sin(u[2])
  13 : Fcn  Expr=-cos(u[1])*sin(u[2])
  21 : Fcn  Expr=-sin(u[3])*cos(u[1])
  22 : Fcn  Expr=cos(u[3])*cos(u[1])
  23 : Fcn
  31 : Fcn  Expr=cos(u[3])*sin(u[2])+sin(u[3])*sin(u[1])*cos(u[2])
  32 : Fcn  Expr=sin(u[3])*sin(u[2])-cos(u[3])*sin(u[1])*cos(u[2])
  33 : Fcn  Expr=cos(u[1])*cos(u[2])
  9x1->3x3 : simulink/Math Operations/Reshape  OutputDimensionality=Customize  OutputDimensions=[3,3]
  Mux2 : Mux  Orientation=down  Inputs=9
  DCM : Outport
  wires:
  9x1->3x3/1 -> DCM/1
  11/1 -> Mux2/1
  21/1 -> Mux2/2
  31/1 -> Mux2/3
  rpw/1 -> 31/1, 21/1, 11/1, 32/1, 22/1, 12/1, 33/1, 23/1, 13/1
  12/1 -> Mux2/4
  22/1 -> Mux2/5
  32/1 -> Mux2/6
  Mux2/1 -> 9x1->3x3/1
  13/1 -> Mux2/7
  23/1 -> Mux2/8
  33/1 -> Mux2/9

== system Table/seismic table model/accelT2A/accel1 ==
  linacc : Inport
  rotacc : Inport  Port=2
  rotvel : Inport  Port=3
  Sum : Sum  Inputs=+++
  crossprod1 : aerospace/Axes Transformations/3x3 cross product
  crossprod2 : aerospace/Axes Transformations/3x3 cross product
  crossprod3 : aerospace/Axes Transformations/3x3 cross product
  dotprod : simulink/Math Operations/Dot Product
  orient : Constant  Value=ea_t(:,id)
  ra_t : Constant  Value=ra_t(:,id)
  out : Outport
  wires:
  orient/1 -> dotprod/2
  dotprod/1 -> out/1
  linacc/1 -> Sum/1
  Sum/1 -> dotprod/1
  rotacc/1 -> crossprod1/1
  ra_t/1 -> crossprod1/2, crossprod2/2
  crossprod1/1 -> Sum/2
  rotvel/1 -> crossprod2/1, crossprod3/1
  crossprod3/1 -> Sum/3
  crossprod2/1 -> crossprod3/2

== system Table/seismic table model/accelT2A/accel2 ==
  linacc : Inport
  rotacc : Inport  Port=2
  rotvel : Inport  Port=3
  Sum : Sum  Inputs=+++
  crossprod1 : aerospace/Axes Transformations/3x3 cross product
  crossprod2 : aerospace/Axes Transformations/3x3 cross product
  crossprod3 : aerospace/Axes Transformations/3x3 cross product
  dotprod : simulink/Math Operations/Dot Product
  orient : Constant  Value=ea_t(:,id)
  ra_t : Constant  Value=ra_t(:,id)
  out : Outport
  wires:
  crossprod2/1 -> crossprod3/2
  crossprod3/1 -> Sum/3
  rotvel/1 -> crossprod3/1, crossprod2/1
  crossprod1/1 -> Sum/2
  ra_t/1 -> crossprod2/2, crossprod1/2
  rotacc/1 -> crossprod1/1
  Sum/1 -> dotprod/1
  linacc/1 -> Sum/1
  dotprod/1 -> out/1
  orient/1 -> dotprod/2

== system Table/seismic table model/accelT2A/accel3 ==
  linacc : Inport
  rotacc : Inport  Port=2
  rotvel : Inport  Port=3
  Sum : Sum  Inputs=+++
  crossprod1 : aerospace/Axes Transformations/3x3 cross product
  crossprod2 : aerospace/Axes Transformations/3x3 cross product
  crossprod3 : aerospace/Axes Transformations/3x3 cross product
  dotprod : simulink/Math Operations/Dot Product
  orient : Constant  Value=ea_t(:,id)
  ra_t : Constant  Value=ra_t(:,id)
  out : Outport
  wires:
  orient/1 -> dotprod/2
  dotprod/1 -> out/1
  linacc/1 -> Sum/1
  Sum/1 -> dotprod/1
  rotacc/1 -> crossprod1/1
  ra_t/1 -> crossprod1/2, crossprod2/2
  crossprod1/1 -> Sum/2
  rotvel/1 -> crossprod2/1, crossprod3/1
  crossprod3/1 -> Sum/3
  crossprod2/1 -> crossprod3/2

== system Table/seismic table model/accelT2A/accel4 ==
  linacc : Inport
  rotacc : Inport  Port=2
  rotvel : Inport  Port=3
  Sum : Sum  Inputs=+++
  crossprod1 : aerospace/Axes Transformations/3x3 cross product
  crossprod2 : aerospace/Axes Transformations/3x3 cross product
  crossprod3 : aerospace/Axes Transformations/3x3 cross product
  dotprod : simulink/Math Operations/Dot Product
  orient : Constant  Value=ea_t(:,id)
  ra_t : Constant  Value=ra_t(:,id)
  out : Outport
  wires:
  crossprod2/1 -> crossprod3/2
  crossprod3/1 -> Sum/3
  rotvel/1 -> crossprod3/1, crossprod2/1
  crossprod1/1 -> Sum/2
  ra_t/1 -> crossprod2/2, crossprod1/2
  rotacc/1 -> crossprod1/1
  Sum/1 -> dotprod/1
  linacc/1 -> Sum/1
  dotprod/1 -> out/1
  orient/1 -> dotprod/2

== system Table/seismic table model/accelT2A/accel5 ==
  linacc : Inport
  rotacc : Inport  Port=2
  rotvel : Inport  Port=3
  Sum : Sum  Inputs=+++
  crossprod1 : aerospace/Axes Transformations/3x3 cross product
  crossprod2 : aerospace/Axes Transformations/3x3 cross product
  crossprod3 : aerospace/Axes Transformations/3x3 cross product
  dotprod : simulink/Math Operations/Dot Product
  orient : Constant  Value=ea_t(:,id)
  ra_t : Constant  Value=ra_t(:,id)
  out : Outport
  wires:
  orient/1 -> dotprod/2
  dotprod/1 -> out/1
  linacc/1 -> Sum/1
  Sum/1 -> dotprod/1
  rotacc/1 -> crossprod1/1
  ra_t/1 -> crossprod1/2, crossprod2/2
  crossprod1/1 -> Sum/2
  rotvel/1 -> crossprod2/1, crossprod3/1
  crossprod3/1 -> Sum/3
  crossprod2/1 -> crossprod3/2

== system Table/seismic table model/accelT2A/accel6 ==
  linacc : Inport
  rotacc : Inport  Port=2
  rotvel : Inport  Port=3
  Sum : Sum  Inputs=+++
  crossprod1 : aerospace/Axes Transformations/3x3 cross product
  crossprod2 : aerospace/Axes Transformations/3x3 cross product
  crossprod3 : aerospace/Axes Transformations/3x3 cross product
  dotprod : simulink/Math Operations/Dot Product
  orient : Constant  Value=ea_t(:,id)
  ra_t : Constant  Value=ra_t(:,id)
  out : Outport
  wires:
  crossprod2/1 -> crossprod3/2
  crossprod3/1 -> Sum/3
  rotvel/1 -> crossprod3/1, crossprod2/1
  crossprod1/1 -> Sum/2
  ra_t/1 -> crossprod2/2, crossprod1/2
  rotacc/1 -> crossprod1/1
  Sum/1 -> dotprod/1
  linacc/1 -> Sum/1
  dotprod/1 -> out/1
  orient/1 -> dotprod/2

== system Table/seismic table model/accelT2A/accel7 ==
  linacc : Inport
  rotacc : Inport  Port=2
  rotvel : Inport  Port=3
  Sum : Sum  Inputs=+++
  crossprod1 : aerospace/Axes Transformations/3x3 cross product
  crossprod2 : aerospace/Axes Transformations/3x3 cross product
  crossprod3 : aerospace/Axes Transformations/3x3 cross product
  dotprod : simulink/Math Operations/Dot Product
  orient : Constant  Value=ea_t(:,id)
  ra_t : Constant  Value=ra_t(:,id)
  out : Outport
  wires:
  orient/1 -> dotprod/2
  dotprod/1 -> out/1
  linacc/1 -> Sum/1
  Sum/1 -> dotprod/1
  rotacc/1 -> crossprod1/1
  ra_t/1 -> crossprod1/2, crossprod2/2
  crossprod1/1 -> Sum/2
  rotvel/1 -> crossprod2/1, crossprod3/1
  crossprod3/1 -> Sum/3
  crossprod2/1 -> crossprod3/2

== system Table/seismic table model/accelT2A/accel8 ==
  linacc : Inport
  rotacc : Inport  Port=2
  rotvel : Inport  Port=3
  Sum : Sum  Inputs=+++
  crossprod1 : aerospace/Axes Transformations/3x3 cross product
  crossprod2 : aerospace/Axes Transformations/3x3 cross product
  crossprod3 : aerospace/Axes Transformations/3x3 cross product
  dotprod : simulink/Math Operations/Dot Product
  orient : Constant  Value=ea_t(:,id)
  ra_t : Constant  Value=ra_t(:,id)
  out : Outport
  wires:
  crossprod2/1 -> crossprod3/2
  crossprod3/1 -> Sum/3
  rotvel/1 -> crossprod3/1, crossprod2/1
  crossprod1/1 -> Sum/2
  ra_t/1 -> crossprod2/2, crossprod1/2
  rotacc/1 -> crossprod1/1
  Sum/1 -> dotprod/1
  linacc/1 -> Sum/1
  dotprod/1 -> out/1
  orient/1 -> dotprod/2

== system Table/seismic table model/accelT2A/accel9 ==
  linacc : Inport
  rotacc : Inport  Port=2
  rotvel : Inport  Port=3
  Sum : Sum  Inputs=+++
  crossprod1 : aerospace/Axes Transformations/3x3 cross product
  crossprod2 : aerospace/Axes Transformations/3x3 cross product
  crossprod3 : aerospace/Axes Transformations/3x3 cross product
  dotprod : simulink/Math Operations/Dot Product
  orient : Constant  Value=ea_t(:,id)
  ra_t : Constant  Value=ra_t(:,id)
  out : Outport
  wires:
  orient/1 -> dotprod/2
  dotprod/1 -> out/1
  linacc/1 -> Sum/1
  Sum/1 -> dotprod/1
  rotacc/1 -> crossprod1/1
  ra_t/1 -> crossprod1/2, crossprod2/2
  crossprod1/1 -> Sum/2
  rotvel/1 -> crossprod2/1, crossprod3/1
  crossprod3/1 -> Sum/3
  crossprod2/1 -> crossprod3/2

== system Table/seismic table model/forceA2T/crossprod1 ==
  A : Inport
  B : Inport  Port=2
  colA : Selector  InputType=Matrix  Elements=[1 3]  Rows=-1  Columns=id  InputPortWidth=3
  colB : Selector  InputType=Matrix  Elements=[1 3]  Rows=-1  Columns=id  InputPortWidth=3
  crossprod : aerospace/Axes Transformations/3x3 cross product
  AxB : Outport
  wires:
  colA/1 -> crossprod/1
  colB/1 -> crossprod/2
  A/1 -> colA/1
  B/1 -> colB/1
  crossprod/1 -> AxB/1

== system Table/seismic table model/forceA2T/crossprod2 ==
  A : Inport
  B : Inport  Port=2
  colA : Selector  InputType=Matrix  Elements=[1 3]  Rows=-1  Columns=id  InputPortWidth=3
  colB : Selector  InputType=Matrix  Elements=[1 3]  Rows=-1  Columns=id  InputPortWidth=3
  crossprod : aerospace/Axes Transformations/3x3 cross product
  AxB : Outport
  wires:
  crossprod/1 -> AxB/1
  B/1 -> colB/1
  A/1 -> colA/1
  colB/1 -> crossprod/2
  colA/1 -> crossprod/1

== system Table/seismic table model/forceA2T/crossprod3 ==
  A : Inport
  B : Inport  Port=2
  colA : Selector  InputType=Matrix  Elements=[1 3]  Rows=-1  Columns=id  InputPortWidth=3
  colB : Selector  InputType=Matrix  Elements=[1 3]  Rows=-1  Columns=id  InputPortWidth=3
  crossprod : aerospace/Axes Transformations/3x3 cross product
  AxB : Outport
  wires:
  colA/1 -> crossprod/1
  colB/1 -> crossprod/2
  A/1 -> colA/1
  B/1 -> colB/1
  crossprod/1 -> AxB/1

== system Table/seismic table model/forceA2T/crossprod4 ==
  A : Inport
  B : Inport  Port=2
  colA : Selector  InputType=Matrix  Elements=[1 3]  Rows=-1  Columns=id  InputPortWidth=3
  colB : Selector  InputType=Matrix  Elements=[1 3]  Rows=-1  Columns=id  InputPortWidth=3
  crossprod : aerospace/Axes Transformations/3x3 cross product
  AxB : Outport
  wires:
  crossprod/1 -> AxB/1
  B/1 -> colB/1
  A/1 -> colA/1
  colB/1 -> crossprod/2
  colA/1 -> crossprod/1

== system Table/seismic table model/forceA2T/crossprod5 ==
  A : Inport
  B : Inport  Port=2
  colA : Selector  InputType=Matrix  Elements=[1 3]  Rows=-1  Columns=id  InputPortWidth=3
  colB : Selector  InputType=Matrix  Elements=[1 3]  Rows=-1  Columns=id  InputPortWidth=3
  crossprod : aerospace/Axes Transformations/3x3 cross product
  AxB : Outport
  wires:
  colA/1 -> crossprod/1
  colB/1 -> crossprod/2
  A/1 -> colA/1
  B/1 -> colB/1
  crossprod/1 -> AxB/1

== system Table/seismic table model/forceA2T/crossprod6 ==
  A : Inport
  B : Inport  Port=2
  colA : Selector  InputType=Matrix  Elements=[1 3]  Rows=-1  Columns=id  InputPortWidth=3
  colB : Selector  InputType=Matrix  Elements=[1 3]  Rows=-1  Columns=id  InputPortWidth=3
  crossprod : aerospace/Axes Transformations/3x3 cross product
  AxB : Outport
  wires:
  crossprod/1 -> AxB/1
  B/1 -> colB/1
  A/1 -> colA/1
  colB/1 -> crossprod/2
  colA/1 -> crossprod/1

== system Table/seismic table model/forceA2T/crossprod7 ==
  A : Inport
  B : Inport  Port=2
  colA : Selector  InputType=Matrix  Elements=[1 3]  Rows=-1  Columns=id  InputPortWidth=3
  colB : Selector  InputType=Matrix  Elements=[1 3]  Rows=-1  Columns=id  InputPortWidth=3
  crossprod : aerospace/Axes Transformations/3x3 cross product
  AxB : Outport
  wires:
  colA/1 -> crossprod/1
  colB/1 -> crossprod/2
  A/1 -> colA/1
  B/1 -> colB/1
  crossprod/1 -> AxB/1

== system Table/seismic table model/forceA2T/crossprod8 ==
  A : Inport
  B : Inport  Port=2
  colA : Selector  InputType=Matrix  Elements=[1 3]  Rows=-1  Columns=id  InputPortWidth=3
  colB : Selector  InputType=Matrix  Elements=[1 3]  Rows=-1  Columns=id  InputPortWidth=3
  crossprod : aerospace/Axes Transformations/3x3 cross product
  AxB : Outport
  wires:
  crossprod/1 -> AxB/1
  B/1 -> colB/1
  A/1 -> colA/1
  colB/1 -> crossprod/2
  colA/1 -> crossprod/1
